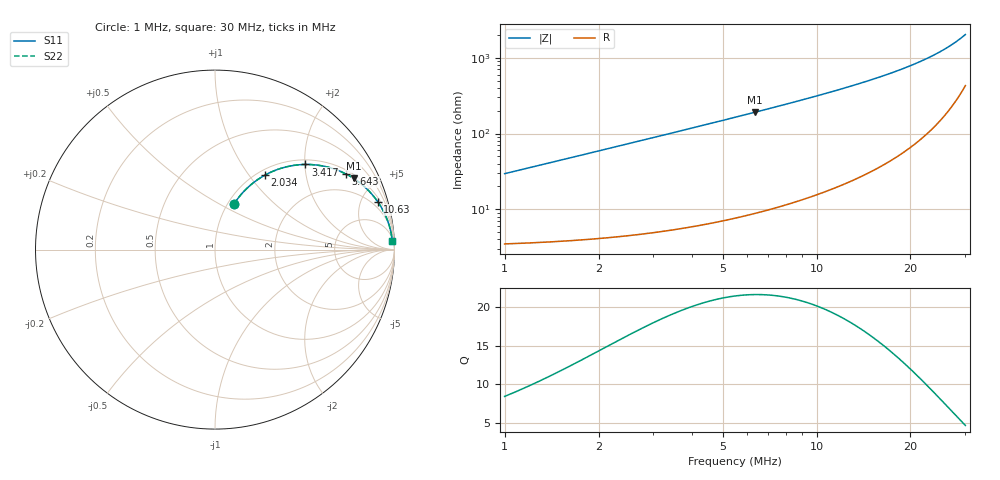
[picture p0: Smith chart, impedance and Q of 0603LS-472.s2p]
# MHz S MA R 50
!Freq  MagS11  AngS11  MagS21  AngS21  MagS12  AngS12  MagS22  AngS22
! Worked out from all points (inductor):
!   801 points, 1 MHz to 30 MHz, reference 50 ohm
!   read as one part in series: L = 4.66 uH near 1.017 MHz
!   highest Q = 21.6 at 6.329 MHz (marker M1), where L = 4.78 uH
!   S11 on the Smith chart (normalised r, x): 1 MHz: 1.07, +0.59; 2.034 MHz: 1.08, +1.19; 3.417 MHz: 1.11, +2.01; 5.643 MHz: 1.16, +3.37; 10.63 MHz: 1.34, +6.70; 30 MHz: 10, +40
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1  0.2743 67.4  0.9298 -15.8  0.9298 -15.8  0.2743 67.4
1.231611  0.3306 65.1  0.9114 -19.2  0.9114 -19.2  0.3306 65.1
1.466142  0.3842 62.5  0.8905 -22.5  0.8905 -22.5  0.3842 62.5
1.73793  0.4417 59.5  0.8639 -26.1  0.8639 -26.1  0.4417 59.5
2.033991  0.4985 56.2  0.8331 -29.8  0.8331 -29.8  0.4985 56.2
2.670046  0.6012 49.7  0.7645 -36.9  0.7645 -36.9  0.6012 49.7
3.416725  0.6923 43.3  0.6862 -43.7  0.6862 -43.7  0.6923 43.3
3.948096  0.7417 39.3  0.6347 -47.8  0.6347 -47.8  0.7417 39.3
4.485179  0.7816 35.9  0.5872 -51.3  0.5872 -51.3  0.7816 35.9
5.052182  0.8153 32.8  0.5419 -54.5  0.5419 -54.5  0.8153 32.8
5.64268  0.8432 30.0  0.4998 -57.4  0.4998 -57.4  0.8432 30.0
5.8379  0.8512 29.1  0.4869 -58.2  0.4869 -58.2  0.8512 29.1
6.329046  0.8688 27.1  0.4567 -60.2  0.4567 -60.2  0.8688 27.1
7.220657  0.8939 24.1  0.4087 -63.2  0.4087 -63.2  0.8939 24.1
8.202926  0.9143 21.3  0.3643 -66.0  0.3643 -66.0  0.9143 21.3
10.63162  0.9453 16.3  0.2818 -70.8  0.2818 -70.8  0.9453 16.3
10.67691  0.9457 16.3  0.2805 -70.8  0.2805 -70.8  0.9457 16.3
12.81861  0.9608 13.2  0.2292 -73.6  0.2292 -73.6  0.9608 13.2
15.52133  0.9721 10.4  0.1811 -76.0  0.1811 -76.0  0.9721 10.4
20.37505  0.9823 6.9  0.1212 -78.2  0.1212 -78.2  0.9823 6.9
25.20106  0.9868 4.5  0.07989 -78.2  0.07989 -78.2  0.9868 4.5
30  0.9886 2.7  0.04874 -75.1  0.04874 -75.1  0.9886 2.7
